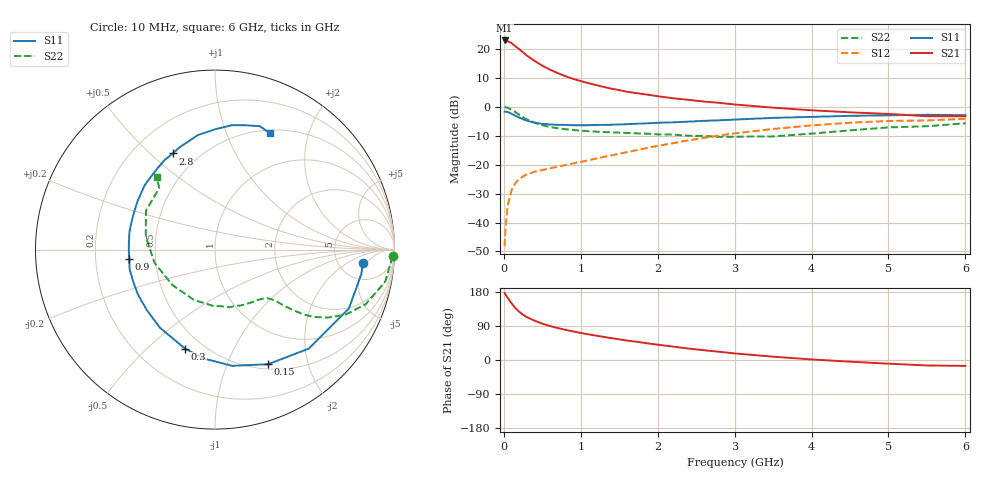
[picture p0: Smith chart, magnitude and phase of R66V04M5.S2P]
! SIEMENS Small Signal Semiconductors
! BFR193
! Si NPN RF Bipolar Junction Transistor in SOT23
! VCE = 6 V  IC = 4.5 mA
! Common Emitter S-Parameters:  May  1996
# GHz  S  MA  R  50
!  f  S11  S21  S12  S22
! GHz  MAG  ANG  MAG  ANG  MAG  ANG  MAG  ANG
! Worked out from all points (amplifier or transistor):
!   36 points, 10 MHz to 6 GHz, reference 50 ohm
!   highest |S21| = 23.0 dB at 10 MHz (marker M1)
!   |S21| within 3 dB of that: start of sweep to 199.7 MHz
!   unconditionally stable (mu >= 1): 947.5 MHz to 1.956 GHz
!   at 250 MHz: K = 0.40, MSG = 21.4 dB, |S12| = -24.0 dB
!   at 1.4 GHz: K = 1.07, MAG = 9.9 dB, |S12| = -16.8 dB
!   at 6 GHz: K = 0.96, MSG = 0.4 dB, |S12| = -4.1 dB
!   S11 on the Smith chart (normalised r, x): 10 MHz: 8.70, -4.07; 150 MHz: 0.56, -1.41; 300 MHz: 0.40, -0.66; 900 MHz: 0.35, -0.05; 2.8 GHz: 0.36, +0.59; 6 GHz: 0.54, +1.44
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0.01  0.828 -5.1  14.08 176.9  0.0039 88.5  0.9926 -2.2
0.02  0.8268 -9.5  13.86 173.3  0.0076 84.0  0.9818 -4.3
0.05  0.8148 -23.7  13.64 164.0  0.0195 78.2  0.9648 -10.7
0.1  0.76 -46.5  12.71 149.5  0.0361 67.5  0.8931 -19.9
0.15  0.704 -65.1  11.17 137.0  0.0483 59.9  0.8115 -26.6
0.2  0.6546 -81.6  9.964 127.3  0.0566 54.4  0.7318 -31.2
0.25  0.6107 -95.6  8.756 119.2  0.0629 50.4  0.6613 -34.5
0.3  0.577 -106.7  7.71 113.1  0.068 48.6  0.6092 -36.3
0.4  0.5327 -125.1  6.23 103.8  0.0756 46.1  0.5345 -38.2
0.5  0.5077 -138.6  5.156 95.9  0.0811 46.3  0.4808 -39.4
0.6  0.4969 -150.0  4.411 89.7  0.0866 46.9  0.4482 -40.1
0.7  0.489 -159.3  3.839 84.4  0.0924 48.5  0.4274 -40.9
0.9  0.4812 -173.8  3.057 75.4  0.105 51.4  0.3983 -42.9
1.1  0.4816 174.0  2.573 67.7  0.1195 54.7  0.3798 -46.3
1.3  0.4884 164.2  2.21 60.9  0.1366 56.8  0.3671 -50.0
1.6  0.5018 151.6  1.83 51.3  0.1648 58.9  0.354 -57.3
2.2  0.5405 131.2  1.409 35.3  0.2358 58.2  0.3312 -75.8
2.8  0.5854 113.7  1.174 21.7  0.3197 52.5  0.3032 -101.8
3.5  0.6452 98.5  0.969 8.8  0.4152 42.2  0.3087 -140.2
4.5  0.6998 82.2  0.805 -4.4  0.5318 25.0  0.3921 169.4
5.5  0.7312 70.1  0.69 -14.4  0.5836 7.5  0.4625 132.2
6  0.7173 64.6  0.688 -15.5  0.6212 2.4  0.5209 128.7
